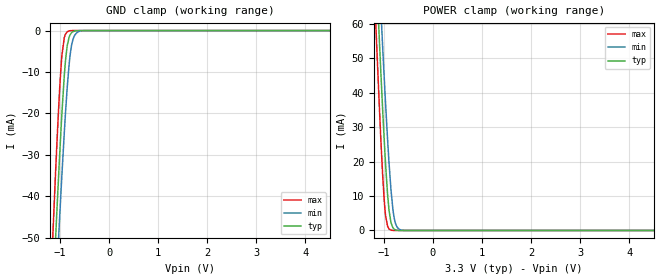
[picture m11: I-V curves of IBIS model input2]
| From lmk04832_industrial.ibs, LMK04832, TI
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|   input2 Model
[Model]   input2
Model_type   Input
Vinl = 0.4
Vinh = 1.2
|   typ   min   max
C_comp   0.3059pF   0.3004pF   0.3116pF
|  Where Nom  PVT is Nominal Process,   3.3V,  25C
|   Fast PVT is Strong Process,   3.45V, -40C
|   Slow PVT is Weak Process,   3.15V, 85C
[Model spec]
|subparameter
Vinl   0.400   0.370   0.430
Vinh   1.200   1.170   1.230
[Voltage Range]   3.3   3.15   3.45
|Junction Temperature
[Temperature Range]   25   85   -40
[Power Clamp Reference]   3.3   3.15   3.45
[GND Clamp Reference]   0   0   0
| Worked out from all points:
|   GND clamp passes 1 mA (typ) near -0.79 V on its own axis
|   POWER clamp passes 1 mA (typ) near -0.82 V on its own axis
[GND Clamp]
|   Voltage   I(typ)   I(min)   I(max)
-3.3V     -672.6mA   -647.6mA   -705.9mA
-1.171V   -70.77mA   -84.12mA   -55.93mA
-1.092V   -50.34mA   -64.75mA   -34.3mA
-1.053V   -40.5mA    -55.3mA    -24.19mA
-1.013V   -31.05mA   -46.07mA   -15.01mA
-963.6mV  -20.09mA   -34.97mA   -6.047mA
-914.1mV  -10.81mA   -24.58mA   -1.675mA
-884.4mV  -6.568mA   -18.87mA   -737.4uA
-815.1mV  -1.569mA   -8.084mA   -73.86uA
-726mV    -198.9uA   -1.756mA   -1.21uA
-547.8mV  -395.6nA   -42.2uA    0A
6.6V      0A         0A         0A
[POWER Clamp]
|   Voltage   I(typ)   I(min)   I(max)
-3.3V     834.5mA    808.2mA    869.6mA
-1.171V   80.81mA    97.58mA    62.55mA
-1.142V   71.18mA    88.41mA    52.4mA
-1.082V   52.44mA    70.4mA     32.99mA
-1.053V   43.42mA    61.61mA    24mA
-1.023V   34.74mA    53.01mA    15.85mA
-963.6mV  18.98mA    36.59mA    4.226mA
-894.3mV  5.851mA    19.62mA    434.7uA
-854.7mV  2.268mA    11.8mA     86.72uA
-765.6mV  185.9uA    2.23mA     1.146uA
-617.1mV  698.1nA    51.77uA    0A
6.6V      0A         0A         0A
